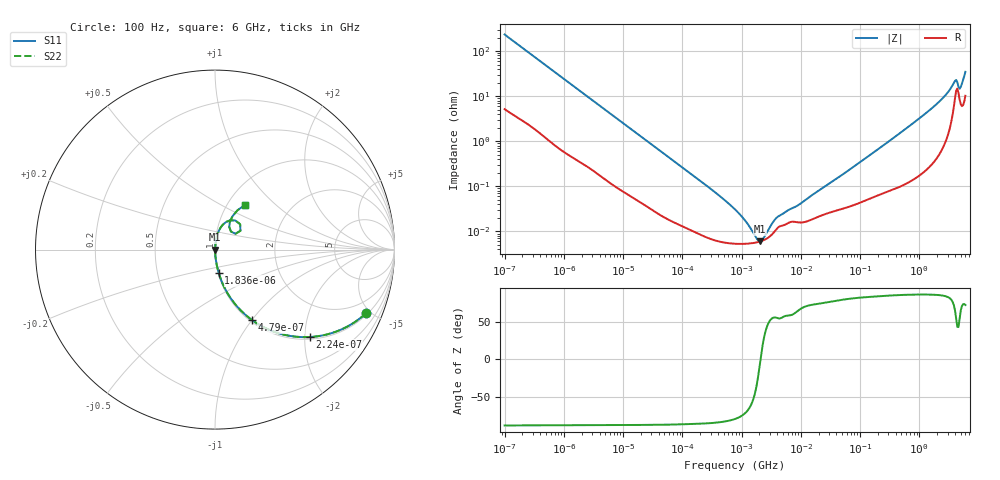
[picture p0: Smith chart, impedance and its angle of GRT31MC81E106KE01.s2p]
!Murata Part Number: GRT31MC81E106KE01
!These Parameters are Measured in Series Mode Connection
!Data Generated on Jun 19, 2026
!  o--ll--o
!Port1  Port2
!  o------o
!Operation Temp=25[degC], DC Bias Voltage=0[V]
!Freq. Start=100[Hz] Stop=6[GHz] 401[Steps]
# Hz S RI R 50
!Freq.(Hz) S11(Real) S11(Imag) S21(Real) S21(Imag) S12(Real) S12(Imag) S22(Real) S22(Imag)
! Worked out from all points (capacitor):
!   401 points, 100 Hz to 6 GHz, reference 50 ohm
!   read as one part in series: C = 6.78 uF near 109 Hz
!   lowest |Z| = 6.01 mohm at 2.074 MHz (marker M1)
!   series resonance near 2.09 MHz, so ESL is about 860 pH
!   S11 on the Smith chart (normalised r, x): 100 Hz: 1.10, -4.67; 224 Hz: 1.05, -2.11; 479 Hz: 1.02, -1.00; 1.836 kHz: 1.01, -0.27; 6 GHz: 1.20, +0.66
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100  0.8399 -0.3559  0.1601 0.3559  0.1601 0.3559  0.8399 -0.3559
224  0.5269 -0.4871  0.4731 0.4871  0.4731 0.4871  0.5269 -0.4871
479  0.2059 -0.3924  0.7941 0.3924  0.7941 0.3924  0.2059 -0.3924
858  0.0787 -0.2578  0.9213 0.2578  0.9213 0.2578  0.0787 -0.2578
1836  0.0207 -0.1298  0.9793 0.1298  0.9793 0.1298  0.0207 -0.1298
2008  0.0177 -0.1192  0.9823 0.1192  0.9823 0.1192  0.0177 -0.1192
6433  0.00261 -0.0387  0.9974 0.0387  0.9974 0.0387  0.00261 -0.0387
40335  0.000281 -0.00641  0.9997 0.00641  0.9997 0.00641  0.000281 -0.00641
316350  6.71e-05 -0.000835  0.9999 0.000835  0.9999 0.000835  6.71e-05 -0.000835
774597  5.33e-05 -0.000304  0.9999 0.000304  0.9999 0.000304  5.33e-05 -0.000304
1516199  5.5e-05 -8.57e-05  0.9999 8.57e-05  0.9999 8.57e-05  5.5e-05 -8.57e-05
2074311  6.01e-05 -2e-06  0.9999 2e-06  0.9999 2e-06  6.01e-05 -2e-06
2713602  7.04e-05 7.01e-05  0.9999 -7.01e-05  0.9999 -7.01e-05  7.04e-05 7.01e-05
4060267  0.00012 0.000173  0.9999 -0.000173  0.9999 -0.000173  0.00012 0.000173
1.555665e7  0.000186 0.000614  0.9998 -0.000614  0.9998 -0.000614  0.000186 0.000614
3.124326e8  0.000888 0.0101  0.9991 -0.0101  0.9991 -0.0101  0.000888 0.0101
1.791126e9  0.00709 0.0594  0.9929 -0.0594  0.9929 -0.0594  0.00709 0.0594
3.065283e9  0.0283 0.1179  0.9717 -0.1179  0.9717 -0.1179  0.0283 0.1179
3.8344e9  0.0848 0.1631  0.9152 -0.1631  0.9152 -0.1631  0.0848 0.1631
4.385646e9  0.1417 0.105  0.8583 -0.105  0.8583 -0.105  0.1417 0.105
5.016141e9  0.0794 0.1263  0.9206 -0.1263  0.9206 -0.1263  0.0794 0.1263
6e9  0.1679 0.2502  0.8321 -0.2502  0.8321 -0.2502  0.1679 0.2502
